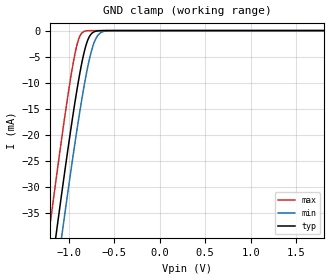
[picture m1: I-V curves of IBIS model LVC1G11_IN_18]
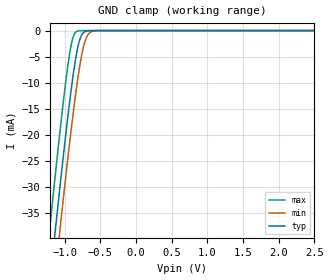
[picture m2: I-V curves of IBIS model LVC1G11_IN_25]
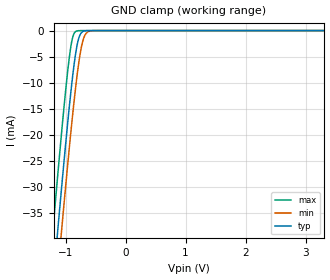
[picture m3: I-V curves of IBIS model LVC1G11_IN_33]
| TEXAS INSTRUMENTS INCORPORATED
| Standard Linear and Logic Group
| IBIS Model of SN74LVC1G11
| SINGLE 3-INPUT POSITIVE-AND GATE
| This file contains package information for the following:
|  SOT 6-pin (DBV) package as [Component] LVC1G11_DBV
|  SOT 6-pin (DCK) package as [Component] LVC1G11_DCK
|  NanoStar WCSP 6-pin (YEP) package as [Component] LVC1G11_YEP
|  NanoFree WCSP 6-pin (YZP) package as [Component] LVC1G11_YZP
| This device can be powered at the following Vccs:
|  1.8 volt Vcc
|  2.5 volt Vcc
|  3.3 volt Vcc
|  5 volt Vcc
| This file provides unique models under the [Model Selector] for each Vcc.
| For operation at a specific Vcc, select the appropriate model after each
| [Model Selector] keyword.
[IBIS Ver]   3.2
[Comment char]  |_char
[File Name]   sn74lvc1g11.ibs
[File Rev]   1.1 | x_die
[Date]   August 30, 2003
[Source]   Data created from TI-SPICE simulations at TI-SLL.
[Notes]   The following is an IBIS list for the SN74LVC1G11.
   Please contact sllibis@ti.com with questions and
   comments concerning SLL IBIS models.
   - Due to the fact that the device is 5.5-V input
   tolerant, the output model has some non-monotonic
   warnings.
   - C_comp values are taken at a different test condition than
   the Ci in data sheet.
   - Power-clamp data has been deleted since there is no
   power-clamp diode in the device.
[Disclaimer] Property of Texas Instruments Incorporated. Unauthorized
   reproduction and/or distribution is strictly prohibited.
   This product is protected under copyright law.
   Created 2002,(C) Copyright 2002, Texas Instruments
   Incorporated, All Rights Reserved
   UNLESS THERE IS A SIGNED, WRITTEN AGREEMENT TO THE
   CONTRARY, TEXAS INSTRUMENTS (TI) IS PROVIDING THE IBIS
   MODELS AND WITHOUT ANY WARRANTY, EXPRESSED OR
   IMPLIED. TI assumes no liability for:
   1) the accuracy of the IBIS models provided to your
   company;
   2) the proper functioning of these IBIS Models in your
   design or for any resulting applications; or
   3) infringement of patents, copyrights or intellectual
   property rights resulting from your use of these IBIS
   models.
   TI provides IBIS Models as a service to our customers.
   You and your company shall not distribute, sell or give
   these models to anyone else without prior written
   permission from TI.
   TI reserves the right to make changes to our products or
   to discontinue any semiconductor product or service
   without notice, and advises our customers to obtain the
   latest version of relevant information to verify, before
   placing orders, that the information being relied on is
   current.
   Please be aware that your receipt and use of the IBIS
   information provided shall serve as acceptance of these
   terms and conditions. If you do not accept these terms,
   you should return or destroy the IBIS models and any
   other accompanying information immediately.
| Component LVC1G11_DBV 6-pin SOT
[Component]   LVC1G11_DBV
[Manufacturer]  Texas Instruments, Inc.
[Package]
|   typ   min   max
R_pkg   2.500e-02   1.900e-02   3.700e-02
L_pkg   1.524e-09   1.260e-09   1.751e-09
C_pkg   2.450e-13   1.980e-13   2.640e-13
[Pin]   signal_name   model_name   R_pin   L_pin   C_pin
1   A   LVC1G11_IN   2.100e-02   1.405e-09   2.460e-13
2   GND   GND   3.700e-02   1.751e-09   2.630e-13
3   B   LVC1G11_IN   2.600e-02   1.493e-09   2.470e-13
4   Y   LVC1G11_OUT   1.900e-02   1.620e-09   2.640e-13
5   VCC   POWER   2.400e-02   1.260e-09   1.980e-13
6   C   LVC1G11_IN   2.100e-02   1.617e-09   2.500e-13
| Component LVC1G11_DCK 6-pin SOT
[Component]   LVC1G11_DCK
[Manufacturer]  Texas Instruments, Inc.
[Package]
|   typ   min   max
R_pkg   1.400e-02   1.100e-02   2.100e-02
L_pkg   9.480e-10   7.840e-10   1.103e-09
C_pkg   1.910e-13   1.670e-13   2.050e-13
[Pin]   signal_name   model_name   R_pin   L_pin   C_pin
1   A   LVC1G11_IN   1.300e-02   9.840e-10   1.960e-13
2   GND   GND   2.100e-02   1.103e-09   2.050e-13
3   B   LVC1G11_IN   1.100e-02   9.980e-10   1.970e-13
4   Y   LVC1G11_OUT   1.300e-02   9.040e-10   1.900e-13
5   VCC   POWER   1.500e-02   7.840e-10   1.670e-13
6   C   LVC1G11_IN   1.200e-02   9.160e-10   1.950e-13
| Component LVC1G11_YEP 6-pin NanoStar WCSP
[Component]   LVC1G11_YEP
[Manufacturer]   Texas Instruments, Inc.
[Package]
|   typ   min   max
R_pkg   0.001   0.001   0.001
L_pkg   1.021nH   1.021nH   1.021nH
C_pkg   0.047pF   0.046pF   0.047pF
[Pin]   signal_name   model_name   R_pin   L_pin   C_pin
1   A   LVC1G11_IN   0.001   0.021nH   0.046pF
2   GND   GND   0.001   0.021nH   0.047pF
3   B   LVC1G11_IN   0.001   0.021nH   0.046pF
4   Y   LVC1G11_OUT   0.001   0.021nH   0.046pF
5   VCC   POWER   0.001   0.021nH   0.047pF
6   C   LVC1G11_IN   0.001   0.021nH   0.046pF
| Component LVC1G11_YZP 6-pin NanoFree WCSP
[Component]   LVC1G11_YZP
[Manufacturer]   Texas Instruments, Inc.
[Package]
|   typ   min   max
R_pkg   0.001   0.001   0.001
L_pkg   1.021nH   1.021nH   1.021nH
C_pkg   0.047pF   0.046pF   0.047pF
[Pin]   signal_name   model_name   R_pin   L_pin   C_pin
1   A   LVC1G11_IN   0.001   0.021nH   0.046pF
2   GND   GND   0.001   0.021nH   0.047pF
3   B   LVC1G11_IN   0.001   0.021nH   0.046pF
4   Y   LVC1G11_OUT   0.001   0.021nH   0.046pF
5   VCC   POWER   0.001   0.021nH   0.047pF
6   C   LVC1G11_IN   0.001   0.021nH   0.046pF
| Model LVC1G11_IN
[Model Selector]   LVC1G11_IN
LVC1G11_IN_18   1.8 volt Vcc
LVC1G11_IN_25   2.5 volt Vcc
LVC1G11_IN_33   3.3 volt Vcc
LVC1G11_IN_50   5 volt Vcc
| Model LVC1G11_OUT
[Model Selector]   LVC1G11_OUT
LVC1G11_OUT_18   1.8 volt Vcc
LVC1G11_OUT_25   2.5 volt Vcc
LVC1G11_OUT_33   3.3 volt Vcc
LVC1G11_OUT_50   5 volt Vcc
| Models and submodels in the file (8): LVC1G11_IN_18 (Input), LVC1G11_IN_25 (Input), LVC1G11_IN_33 (Input), LVC1G11_IN_50 (Input), LVC1G11_OUT_18 (Output), LVC1G11_OUT_25 (Output), LVC1G11_OUT_33 (Output), LVC1G11_OUT_50 (Output)
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[Model]   LVC1G11_IN_18
Model_type  Input
Vinl=0.5775
Vinh=1.2675
| variable   typ   min   max
C_comp   3.63pF   3.10pF   4.42pF
[Temperature Range]   40   100   -40
| Ambient temperature   25   85   -40
[Voltage range]   1.8   1.65   1.95
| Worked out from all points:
|   GND clamp passes 1 mA (typ) near -0.77 V on its own axis
[GND Clamp]
| LVC1G11_IN_18
|   Voltage   I(typ)   I(min)   I(max)
-5.5V     -655.2mA   -662.2mA   -646.6mA
-1.215V   -49.6mA    -57.88mA   -38.96mA
-1.135V   -39.07mA   -47.36mA   -28.42mA
-1.075V   -31.35mA   -39.6mA    -20.75mA
-1.055V   -28.82mA   -37.05mA   -18.27mA
-955mV    -16.68mA   -24.66mA   -6.874mA
-885mV    -9.098mA   -16.55mA   -1.486mA
-825mV    -3.922mA   -10.26mA   -137.1uA
-780mV    -1.472mA   -6.227mA   -17.15uA
-715mV    -205.4uA   -2.128mA   -808.5nA
-650mV    -22.01uA   -443.9uA   -37.93nA
1.8V      3.326pA    6.142pA    3.026pA
[Model]   LVC1G11_IN_25
Model_type  Input
Vinl=0.7
Vinh=1.7
| variable   typ   min   max
C_comp   3.56pF   2.89pF   4.51pF
[Temperature Range]   40   100   -40
| Ambient temperature   25   85   -40
[Voltage range]   2.5   2.3   2.7
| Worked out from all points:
|   GND clamp passes 1 mA (typ) near -0.77 V on its own axis
[GND Clamp]
| LVC1G11_IN_25
|   Voltage   I(typ)   I(min)   I(max)
-5.5V     -655.2mA   -662.2mA   -646.6mA
-1.215V   -49.6mA    -57.88mA   -38.96mA
-1.14V    -39.72mA   -48.01mA   -29.07mA
-1.12V    -37.12mA   -45.41mA   -26.48mA
-1.08V    -31.98mA   -40.25mA   -21.38mA
-1.06V    -29.44mA   -37.69mA   -18.89mA
-960mV    -17.26mA   -25.26mA   -7.377mA
-890mV    -9.597mA   -17.1mA    -1.734mA
-785mV    -1.671mA   -6.635mA   -21.67uA
-720mV    -242.5uA   -2.354mA   -1.023uA
-650mV    -22.01uA   -443.9uA   -37.93nA
2.5V      4.713pA    7.577pA    4.389pA
[Model]   LVC1G11_IN_33
Model_type  Input
Vinl=0.8
Vinh=2.0
| variable   typ   min   max
C_comp   3.49pF   2.77pF   4.54pF
[Temperature Range]   40   100   -40
| Ambient temperature   25   85   -40
[Voltage range]   3.3   3   3.6
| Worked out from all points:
|   GND clamp passes 1 mA (typ) near -0.77 V on its own axis
[GND Clamp]
| LVC1G11_IN_33
|   Voltage   I(typ)   I(min)   I(max)
-5.5V     -655.2mA   -662.2mA   -646.6mA
-1.225V   -50.93mA   -59.21mA   -40.3mA
-1.145V   -40.37mA   -48.66mA   -29.72mA
-1.12V    -37.12mA   -45.41mA   -26.48mA
-1.08V    -31.98mA   -40.25mA   -21.38mA
-1.06V    -29.44mA   -37.69mA   -18.89mA
-965mV    -17.84mA   -25.87mA   -7.89mA
-885mV    -9.098mA   -16.55mA   -1.486mA
-780mV    -1.472mA   -6.227mA   -17.15uA
-715mV    -205.4uA   -2.128mA   -808.5nA
-640mV    -15.53uA   -338.1uA   -23.69nA
3.3V      6.304pA    9.258pA    5.93pA
